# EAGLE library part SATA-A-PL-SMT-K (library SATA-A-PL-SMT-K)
Conn SATA PL 7 POS 1.27mm Solder RA SMD 7 Terminal 1 Port Tray/Tube Source: Datasheet
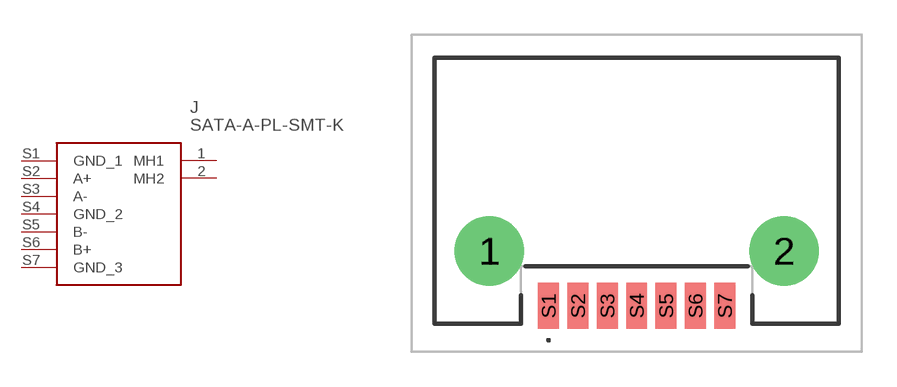
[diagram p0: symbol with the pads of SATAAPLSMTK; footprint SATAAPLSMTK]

Designator prefix J

## SATA-A-PL-SMT-K (Description: Conn SATA PL 7 POS 1.27mm Solder RA SMD 7 Terminal 1 Port Tray/Tube; Height: 5.8928mm; Manufacturer_Name: Adam Tech; Manufacturer_Part_Number: SATA-A-PL-SMT-K; Mouser_Part_Number: 737-SATA-A-PL-SMT-K; Mouser_Price-Stock: https://www.mouser.co.uk/ProductDetail/Adam-Tech/SATA-A-PL-SMT-K?qs=HoCaDK9Nz5dztr92%2FSCAMw%3D%3D)  [SATAAPLSMTK]
1  MH1
2  MH2
S1  GND_1
S2  A+
S3  A-
S4  GND_2
S5  B-
S6  B+
S7  GND_3

## Footprint SATAAPLSMTK (pad centres in mm)
SATA-A-PL-SMT-K-3
drill 1.5 pad 3: 1 -6.37,-2.6; 2 6.37,-2.6
smd 0.9 x 2: S1 -3.81,-4.96; S2 -2.54,-4.96; S3 -1.27,-4.96; S4 0,-4.96; S5 1.27,-4.96; S6 2.54,-4.96; S7 3.81,-4.96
